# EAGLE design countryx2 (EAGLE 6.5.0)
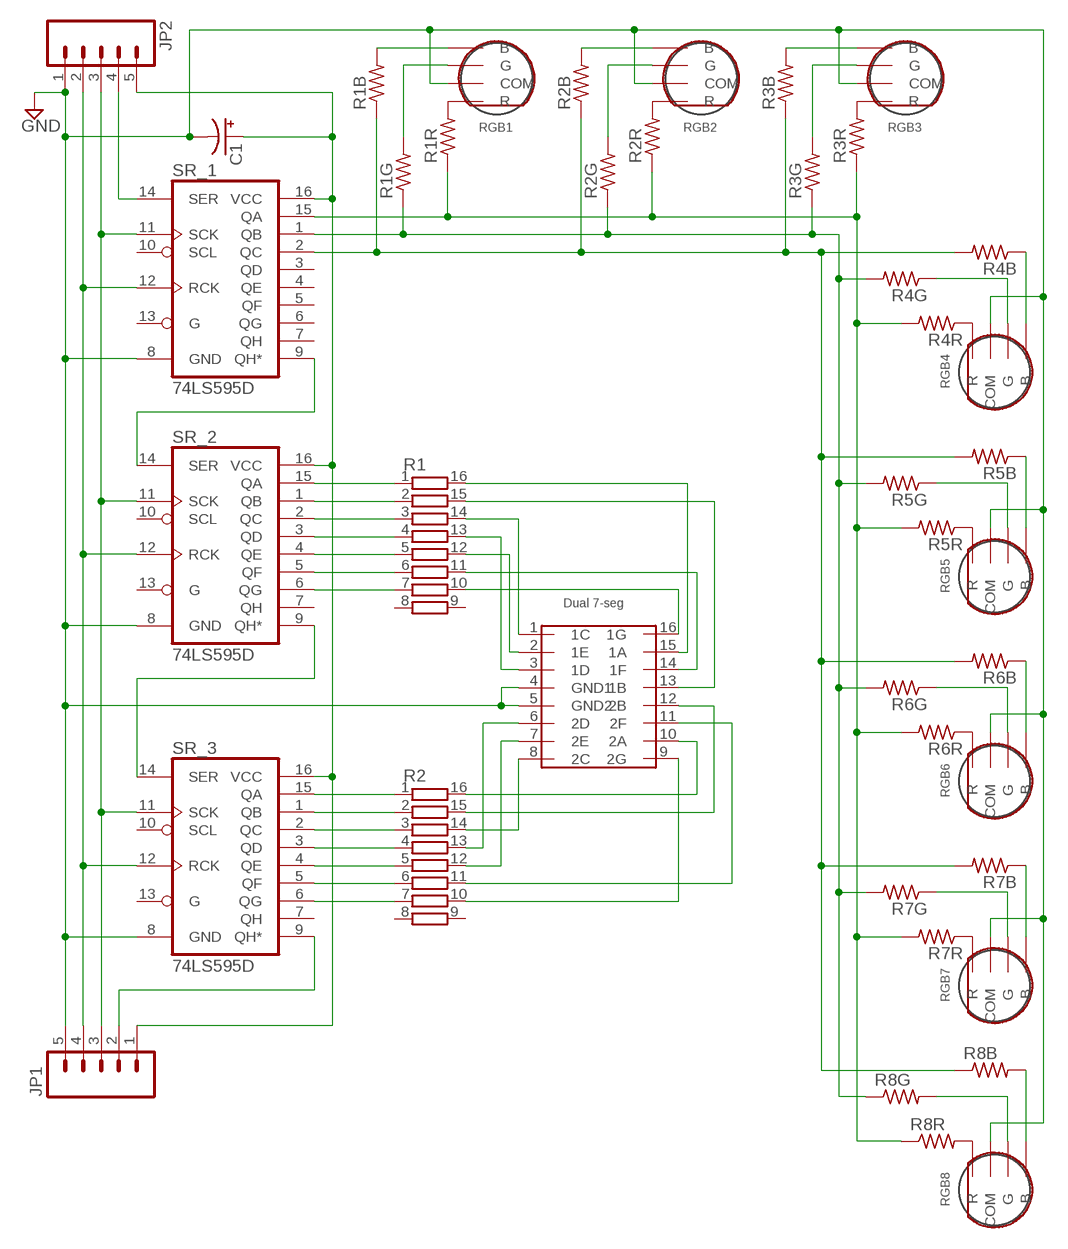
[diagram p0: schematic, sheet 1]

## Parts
C1  CPOL-USE2,5-6E  [E2,5-6E]
JP1  M05LOCK  [1X05_LOCK]
JP2  M05LOCK  [1X05_LOCK]
R1  4816P-T01  [4816P]
R1B  R-US_M0805  [M0805]
R1G  R-US_M0805  [M0805]
R1R  R-US_M0805  [M0805]
R2  4816P-T01  [4816P]
R2B  R-US_M0805  [M0805]
R2G  R-US_M0805  [M0805]
R2R  R-US_M0805  [M0805]
R3B  R-US_M0805  [M0805]
R3G  R-US_M0805  [M0805]
R3R  R-US_M0805  [M0805]
R4B  R-US_M0805  [M0805]
R4G  R-US_M0805  [M0805]
R4R  R-US_M0805  [M0805]
R5B  R-US_M0805  [M0805]
R5G  R-US_M0805  [M0805]
R5R  R-US_M0805  [M0805]
R6B  R-US_M0805  [M0805]
R6G  R-US_M0805  [M0805]
R6R  R-US_M0805  [M0805]
R7B  R-US_M0805  [M0805]
R7G  R-US_M0805  [M0805]
R7R  R-US_M0805  [M0805]
R8B  R-US_M0805  [M0805]
R8G  R-US_M0805  [M0805]
R8R  R-US_M0805  [M0805]
RGB1  RGBLED  [3LED]
RGB2  RGBLED  [3LED]
RGB3  RGBLED  [3LED]
RGB4  RGBLED  [3LED]
RGB5  RGBLED  [3LED]
RGB6  RGBLED  [3LED]
RGB7  RGBLED  [3LED]
RGB8  RGBLED  [3LED]
SR_1  74LS595D  [SO16]
SR_2  74LS595D  [SO16]
SR_3  74LS595D  [SO16]
U$1  HDSP-G03E  [HDSP-G]

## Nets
GND: C1.- JP1.5 JP2.1 RGB1.COM RGB2.COM RGB3.COM RGB4.COM RGB5.COM RGB6.COM RGB7.COM RGB8.COM SR_1.8(GND) SR_2.8(GND) SR_3.8(GND) U$1.4(GND1) U$1.5(GND2)
N$1: R1R.1 R2R.1 R3R.1 R4R.2 R5R.2 R6R.2 R7R.2 R8R.1 SR_1.15(QA)
N$2: R1B.1 R2B.1 R3B.1 R4B.2 R5B.2 R6B.2 R7B.2 R8B.1 SR_1.2(QC)
N$3: R8R.2 RGB8.R
N$4: R1.10 U$1.16(1G)
N$5: R1.11 U$1.14(1F)
N$6: R1.14 U$1.1(1C)
N$7: R1.7 SR_2.6(QG)
N$8: R1R.2 RGB1.R
N$9: R1.16 U$1.15(1A)
N$10: R1.15 U$1.13(1B)
N$11: R2.15 U$1.12(2B)
N$12: R2.11 U$1.11(2F)
N$13: R2.2 SR_3.1(QB)
N$14: R2.13 U$1.6(2D)
N$15: R2.1 SR_3.15(QA)
N$16: R1.4 SR_2.3(QD)
N$17: R2.12 U$1.7(2E)
N$18: R2R.2 RGB2.R
N$19: R2.3 SR_3.2(QC)
N$20: R3R.2 RGB3.R
N$21: R2.16 U$1.10(2A)
N$22: R2.4 SR_3.3(QD)
N$23: R2.5 SR_3.4(QE)
N$24: R2.6 SR_3.5(QF)
N$25: R1G.2 RGB1.G
N$26: R2G.2 RGB2.G
N$27: R3G.2 RGB3.G
N$28: R1B.2 RGB1.B
N$29: R2B.2 RGB2.B
N$30: R3B.2 RGB3.B
N$31: R2.7 SR_3.6(QG)
N$32: R1G.1 R2G.1 R3G.1 R4G.2 R5G.2 R6G.2 R7G.2 R8G.1 SR_1.1(QB)
N$33: R1.5 SR_2.4(QE)
N$34: R4G.1 RGB4.G
N$35: R4B.1 RGB4.B
N$36: R4R.1 RGB4.R
N$37: R2.10 U$1.9(2G)
N$38: R1.12 U$1.2(1E)
N$39: R5G.1 RGB5.G
N$40: R5B.1 RGB5.B
N$41: R5R.1 RGB5.R
N$42: R1.6 SR_2.5(QF)
N$43: R6G.1 RGB6.G
N$44: R6B.1 RGB6.B
N$45: R6R.1 RGB6.R
N$46: R8G.2 RGB8.G
N$47: R8B.2 RGB8.B
N$48: R1.13 U$1.3(1D)
N$49: R7G.1 RGB7.G
N$50: R7B.1 RGB7.B
N$51: R7R.1 RGB7.R
N$52: R2.14 U$1.8(2C)
N$53: R1.3 SR_2.2(QC)
N$54: R1.2 SR_2.1(QB)
N$55: R1.1 SR_2.15(QA)
RCLK: JP1.4 JP2.2 SR_1.12(RCK) SR_2.12(RCK) SR_3.12(RCK)
SCLK: JP1.3 JP2.3 SR_1.11(SCK) SR_2.11(SCK) SR_3.11(SCK)
SER_12: SR_1.9(QH*) SR_2.14(SER)
SER_23: SR_2.9(QH*) SR_3.14(SER)
SER_IN: JP2.4 SR_1.14(SER)
SER_OUT: JP1.2 SR_3.9(QH*)
VCC: C1.+ JP1.1 JP2.5 SR_1.16(VCC) SR_2.16(VCC) SR_3.16(VCC)
Unconnected: R1.8 R1.9 R2.8 R2.9 SR_1.3(QD) SR_1.4(QE) SR_1.5(QF) SR_1.6(QG) SR_1.7(QH) SR_1.10(SCL) SR_1.13(G) SR_2.7(QH) SR_2.10(SCL) SR_2.13(G) SR_3.7(QH) SR_3.10(SCL) SR_3.13(G)

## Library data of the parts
C1 = Power Supply:CPOL-US: POLARIZED CAPACITOR, American symbol
JP1 JP2 = SparkFun-Connectors:M05: Header 5 Standard 5-pin 0.1" header. Use with straight break away headers (SKU : PRT-00116), right angle break away headers (PRT-00553), swiss pins (PRT-00743), machine pins (PRT-00117), and female headers (PRT-00115). Molex polarized connector foot print use with SKU : PRT-08230 with associated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
R1 R2 = resistor-bourns:4816P-T01: BOURNS RESISTOR NETWORK; MF: BOURNS, INC.; MPN: 4816P-T01-684LF; OC_FARNELL: 9357483; OC_NEWARK: 33K0707
R1B R1G R1R R2B R2G R2R R3B R3G R3R R4B R4G R4R R5B R5G R5R R6B R6G R6R R7B R7G R7R R8B R8G R8R = resistor:R-US_: RESISTOR, American symbol
RGB1-RGB8 = RISK:RGBLED
SR_1-SR_3 = SparkFun-DigitalIC:74*595: 8-bit SHIFT REGISTER, output latch; PROD_ID: IC-07875
U$1 = RISK:HDSP-G03E

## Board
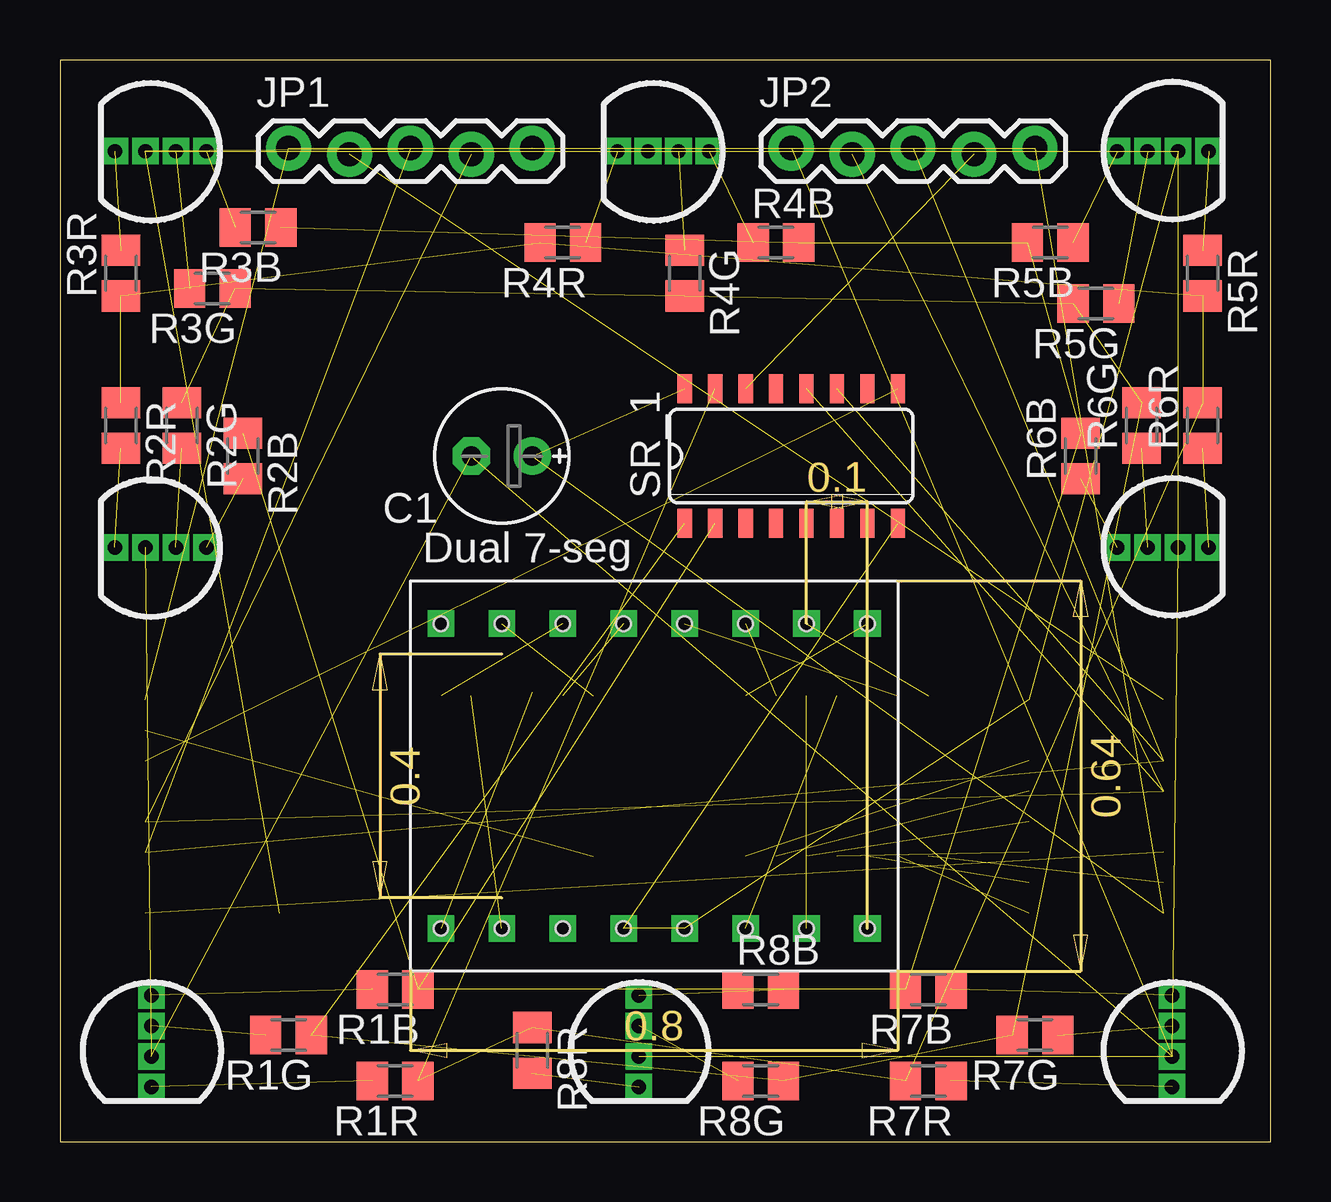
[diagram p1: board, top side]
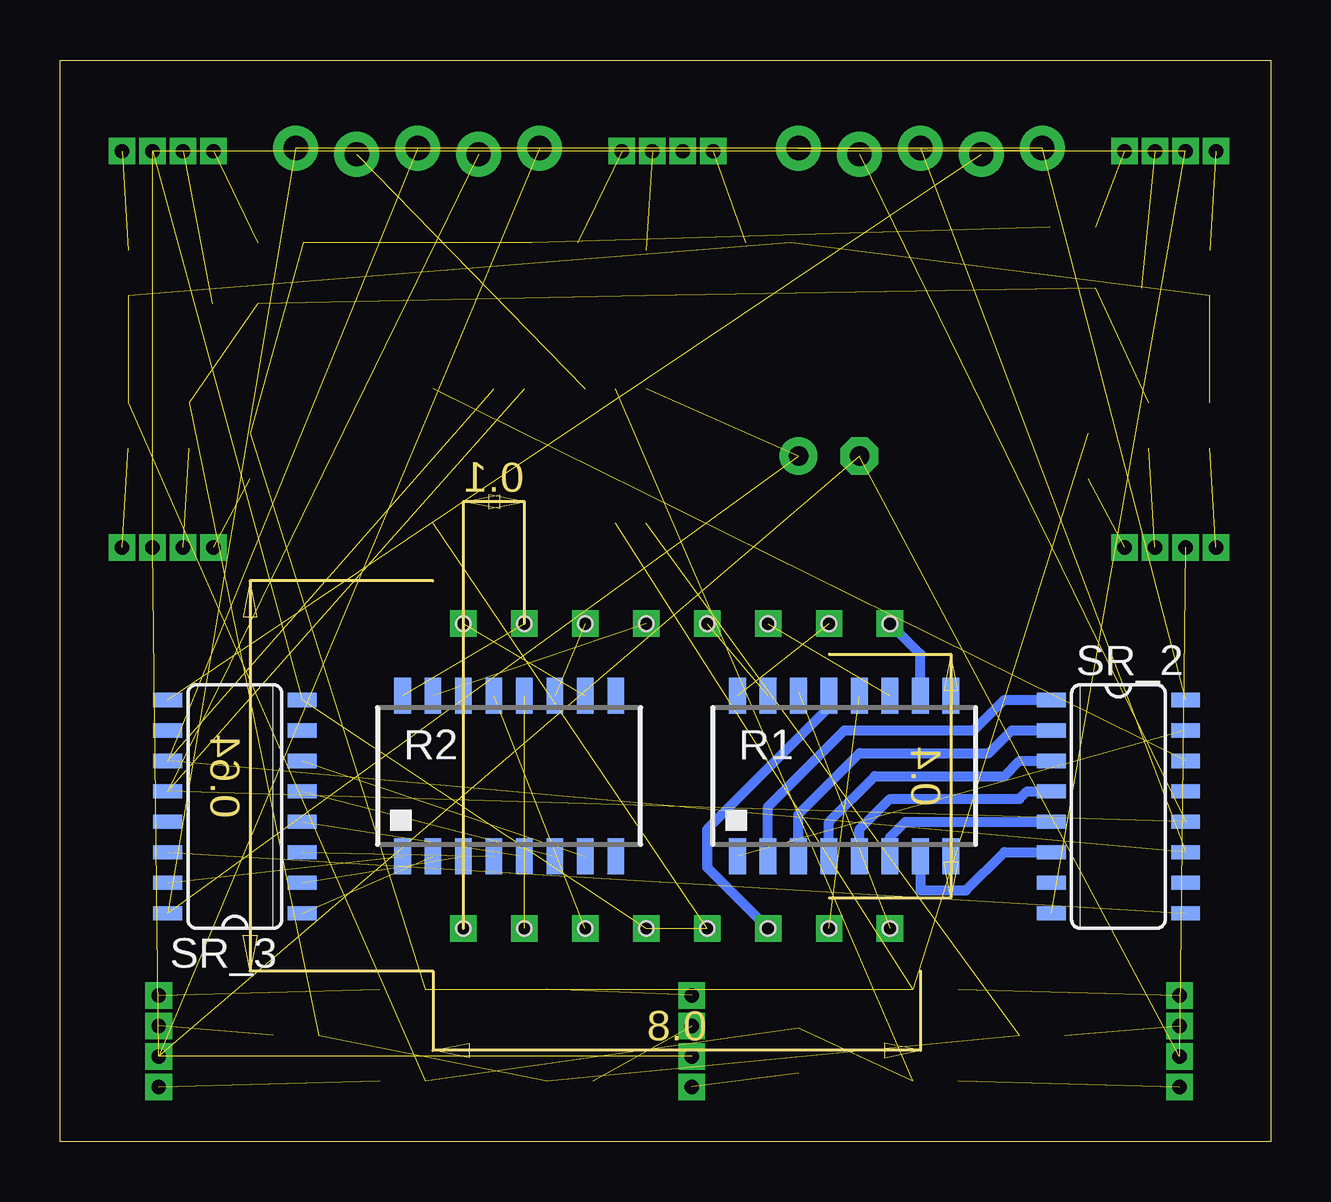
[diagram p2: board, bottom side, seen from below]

Size 50.47 x 45.08 mm. Coordinates in mm from the lower left corner, seen from the top.
Outline: 0,0 50.47,0 50.47,45.08 0,45.08 0,0
Copper layers (1*16): Top 0.035mm / dielectric 1.5mm / Bottom 0.035mm
Design rules "default": minimum track width 10mil, minimum drill 24mil, track to track 8mil, track to pad 8mil, pad to pad 8mil, via to via 8mil, smd to smd 8mil, copper to edge 40mil, drill to drill 8mil, minimum pad ring 10mil, minimum via ring 8mil, stop-mask expansion 4mil, vias tented up to drill 0mil, thermal gap 10mil

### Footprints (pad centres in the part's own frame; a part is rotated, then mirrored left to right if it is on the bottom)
E2,5-6E = drill 0.813 pad 1.575: + -1.27,0 | drill 0.813 pad 1.575 octagon: - 1.27,0
1X05_LOCK = drill 1.016 pad 1.88: 1 0,0.127; 2 2.54,-0.127; 3 5.08,0.127; 4 7.62,-0.127; 5 10.16,0.127
4816P = smd 0.7 x 1.5: 1 -4.445,-3.346; 2 -3.175,-3.346; 3 -1.905,-3.346; 4 -0.635,-3.346; 5 0.635,-3.346; 6 1.905,-3.346; 7 3.175,-3.346; 8 4.445,-3.346; 9 4.445,3.346; 10 3.175,3.346; 11 1.905,3.346; 12 0.635,3.346; 13 -0.635,3.346; 14 -1.905,3.346; 15 -3.175,3.346; 16 -4.445,3.346
M0805 = smd 1.3 x 1.6: 1 -0.95,0; 2 0.95,0
3LED = drill 0.6 pad 0.61 square: B 0,2.286; COM 0,-0.254; G 0,1.016; R 0,-1.524
SO16 = smd 0.6 x 1.2: 1 -4.445,-2.8; 2 -3.175,-2.8; 3 -1.905,-2.8; 4 -0.635,-2.8; 5 0.635,-2.8; 6 1.905,-2.8; 7 3.175,-2.8; 8 4.445,-2.8; 9 4.445,2.8; 10 3.175,2.8; 11 1.905,2.8; 12 0.635,2.8; 13 -0.635,2.8; 14 -1.905,2.8; 15 -3.175,2.8; 16 -4.445,2.8
HDSP-G = drill 0.6 square: 1 -8.89,-6.35; 2 -6.35,-6.35; 3 -3.81,-6.35; 4 -1.27,-6.35; 5 1.27,-6.35; 6 3.81,-6.35; 7 6.35,-6.35; 8 8.89,-6.35; 9 8.89,6.35; 10 6.35,6.35; 11 3.81,6.35; 12 1.27,6.35; 13 -1.27,6.35; 14 -3.81,6.35; 15 -6.35,6.35; 16 -8.89,6.35 | hole 0.6: 1.27,-6.35; 1.27,-6.35; 1.27,-6.35; 1.27,-6.35; -1.27,-6.35; -1.27,-6.35; -3.81,-6.35; -3.81,-6.35; -6.35,-6.35; -6.35,-6.35; -6.35,-6.35; -8.89,-6.35; -8.89,-6.35; 3.81,-6.35; 3.81,-6.35; 3.81,-6.35; 6.35,-6.35; 6.35,-6.35; 8.89,-6.35; 8.89,-6.35; 8.89,-6.35; 8.89,6.35; 8.89,6.35; 6.35,6.35; 6.35,6.35; 3.81,6.35; 3.81,6.35; 1.27,6.35; 1.27,6.35; -1.27,6.35; -1.27,6.35; -3.81,6.35; -3.81,6.35; -6.35,6.35; -6.35,6.35; -6.35,6.35; -8.89,6.35; -8.89,6.35

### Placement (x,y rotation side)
C1  18.41,28.57 180 top
JP1  9.53,41.27 0 top
JP2  30.48,41.27 0 top
R1  17.78,15.24 0 bottom
R1B  13.97,6.35 180 top
R1G  9.53,4.45 180 top
R1R  13.97,2.54 180 top
R2  31.75,15.24 0 bottom
R2B  7.62,28.57 270 top
R2G  5.08,29.84 270 top
R2R  2.54,29.84 270 top
R3B  8.26,38.1 180 top
R3G  6.35,35.56 180 top
R3R  2.54,36.2 90 top
R4B  29.84,37.47 0 top
R4G  26.04,36.2 270 top
R4R  20.95,37.47 180 top
R5B  41.27,37.47 180 top
R5G  43.18,34.92 180 top
R5R  47.62,36.2 270 top
R6B  42.55,28.57 90 top
R6G  45.09,29.84 90 top
R6R  47.62,29.84 90 top
R7B  36.2,6.35 180 top
R7G  40.64,4.45 180 top
R7R  36.2,2.54 180 top
R8B  29.21,6.35 0 top
R8G  29.21,2.54 180 top
R8R  19.68,3.81 270 top
RGB1  3.81,3.81 0 top
RGB2  3.81,24.77 270 top
RGB3  3.81,41.27 270 top
RGB4  24.77,41.27 270 top
RGB5  46.35,41.27 90 top
RGB6  46.35,24.77 90 top
RGB7  46.35,3.81 0 top
RGB8  24.13,3.81 0 top
SR_1  30.48,28.57 0 top
SR_2  6.35,13.97 270 bottom
SR_3  43.18,13.97 90 bottom
U$1  24.77,15.24 0 top

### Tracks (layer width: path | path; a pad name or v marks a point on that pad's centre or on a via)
GND  (15 unrouted)
N$1  (8 unrouted)
N$2  (8 unrouted)
N$3  (1 unrouted)
N$4
  Bottom 0.406: R1.10 14.61,20.32 U$1.16
N$5  (1 unrouted)
N$6  (1 unrouted)
  Bottom 0.406: R1.14 19.68,18.73
N$7
  Bottom 0.406: R1.7 14.61,10.48 12.7,10.48 11.11,12.06 SR_2.6
N$8  (1 unrouted)
N$9  (1 unrouted)
N$10  (1 unrouted)
N$11  (1 unrouted)
N$12  (1 unrouted)
N$13  (1 unrouted)
N$14  (1 unrouted)
N$15  (1 unrouted)
N$16
  Bottom 0.406: R1.4 18.41,13.34 16.51,15.24 11.11,15.24 10.48,15.88 SR_2.3
N$17  (1 unrouted)
N$18  (1 unrouted)
N$19  (1 unrouted)
N$20  (1 unrouted)
N$21  (1 unrouted)
N$22  (1 unrouted)
N$23  (1 unrouted)
N$24  (1 unrouted)
N$25  (1 unrouted)
N$26  (1 unrouted)
N$27  (1 unrouted)
N$28  (1 unrouted)
N$29  (1 unrouted)
N$30  (1 unrouted)
N$31  (1 unrouted)
N$32  (8 unrouted)
N$33
  Bottom 0.406: R1.5 17.14,13.02 15.88,14.29 10.48,14.29 10.16,14.61 SR_2.4
N$34  (1 unrouted)
N$35  (1 unrouted)
N$36  (1 unrouted)
N$37  (1 unrouted)
N$38  (1 unrouted)
N$39  (1 unrouted)
N$40  (1 unrouted)
N$41  (1 unrouted)
N$42
  Bottom 0.406: R1.6 15.88,12.7 15.24,13.34 SR_2.5
N$43  (1 unrouted)
N$44  (1 unrouted)
N$45  (1 unrouted)
N$46  (1 unrouted)
N$47  (1 unrouted)
N$48
  Bottom 0.406: R1.13 18.41,18.1 23.5,13.02 23.5,11.43 U$1.3
N$49  (1 unrouted)
N$50  (1 unrouted)
N$51  (1 unrouted)
N$52  (1 unrouted)
N$53
  Bottom 0.406: R1.3 19.68,13.65 17.14,16.19 11.75,16.19 10.79,17.14 SR_2.2
N$54
  Bottom 0.406: R1.2 20.95,13.97 17.78,17.14 12.38,17.14 11.11,18.41 SR_2.1
N$55  (1 unrouted)
RCLK  (4 unrouted)
SCLK  (4 unrouted)
SER_12  (1 unrouted)
SER_23  (1 unrouted)
SER_IN  (1 unrouted)
SER_OUT  (1 unrouted)
VCC  (5 unrouted)

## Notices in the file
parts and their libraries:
SparkFun-DigitalIC: Licensing: Creative Commons ShareAlike 4.0 International - https://creativecommons.org/licenses/by-sa/4.0
